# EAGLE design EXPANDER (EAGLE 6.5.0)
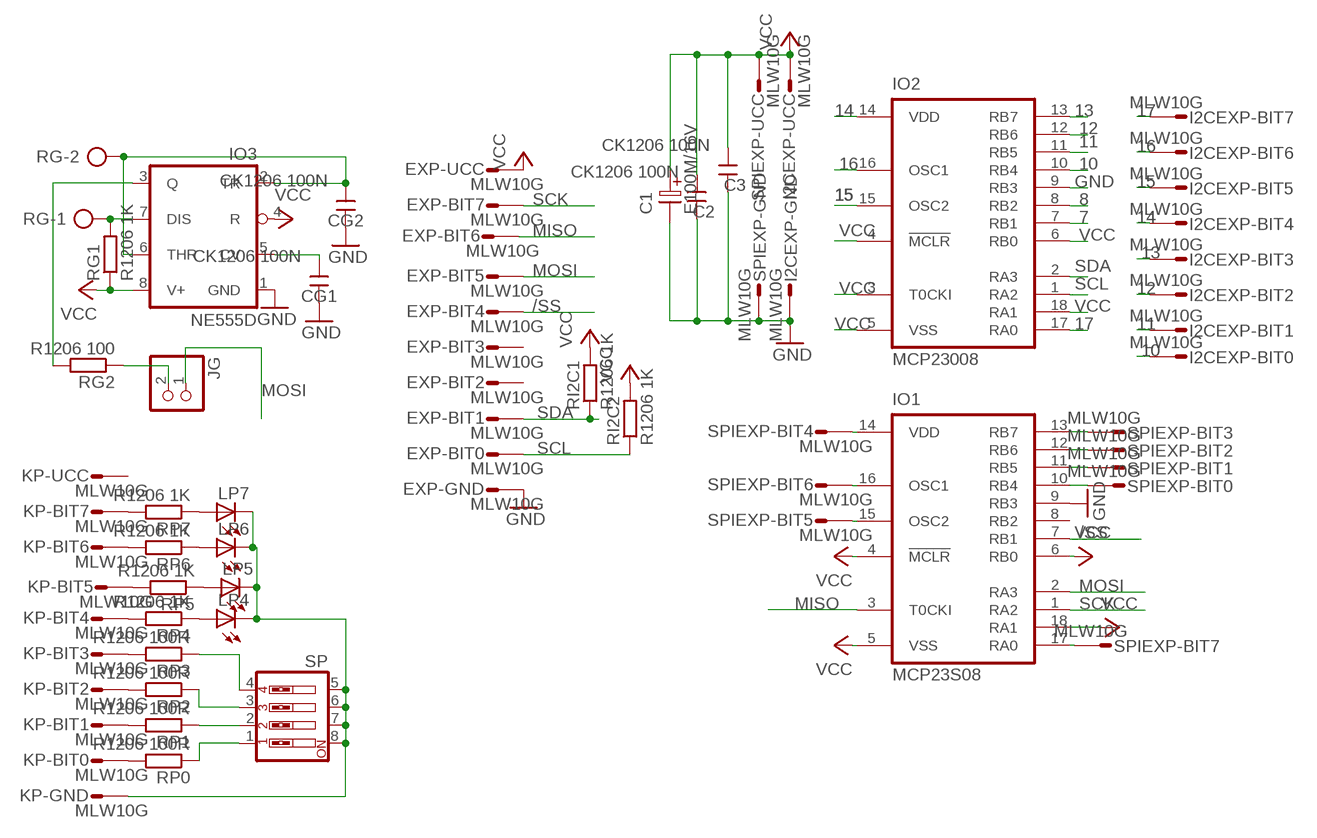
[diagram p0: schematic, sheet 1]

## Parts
C1  E100M/16V  CEL2,5  [ES-2,5L]
C2  CK1206 100N  CK+  [CK+]
C3  CK1206 100N  CK+  [CK+]
CG1  CK1206 100N  CK+  [CK+]
CG2  CK1206 100N  CK+  [CK+]
EXP  MLW10G  PSL10MLW10G  [MLW10G]
I2CEXP  MLW10G  PSL10MLW10G  [MLW10G]
IO1  MCP23S08  PIC16C710SO  [SO-18W]
IO2  MCP23008  PIC16C710SO  [SO-18W]
IO3  NE555D  [SO08]
JG  PINHD-1X2  [1X02]
KP  MLW10G  PSL10MLW10G  [MLW10G]
LP4  LED3MM  [LED3MM]
LP5  LED3MM  [LED3MM]
LP6  LED3MM  [LED3MM]
LP7  LED3MM  [LED3MM]
RG  AK500/2  [AK500/2]
RG1  R1206 1K  R-EU_R1206  [R1206]
RG2  R1206 100  R-EU_R1206  [R1206]
RI2C1  R1206 1K  R-EU_R1206  [R1206]
RI2C2  R1206 1K  R-EU_R1206  [R1206]
RP0  R1206 100R  R-EU_R1206  [R1206]
RP1  R1206 100R  R-EU_R1206  [R1206]
RP2  R1206 100R  R-EU_R1206  [R1206]
RP3  R1206 100R  R-EU_R1206  [R1206]
RP4  R1206 1K  R-EU_R1206  [R1206]
RP5  R1206 1K  R-EU_R1206  [R1206]
RP6  R1206 1K  R-EU_R1206  [R1206]
RP7  R1206 1K  R-EU_R1206  [R1206]
SP  SW_DIP-4  [EDG-04]
SPIEXP  MLW10G  PSL10MLW10G  [MLW10G]
U$1  RAM  [RAM]

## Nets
7: IO2.7(RB1)
8: IO2.8(RB2)
10: I2CEXP.9 IO2.10(RB4)
11: I2CEXP.8 IO2.11(RB5)
12: I2CEXP.7 IO2.12(RB6)
13: I2CEXP.6 IO2.13(RB7)
14: I2CEXP.5 IO2.14(VDD)
15: I2CEXP.4 IO2.15(OSC2)
16: I2CEXP.3 IO2.16(OSC1)
17: I2CEXP.2 IO2.17(RA0)
/SS: EXP.5 IO1.7(RB1)
GND: C1.2 C2.1 C3.1 CG1.1 CG2.1 EXP.10 I2CEXP.10 IO1.9(RB3) IO2.9(RB3) IO3.1(GND) SPIEXP.10
MISO: EXP.3 IO1.3(T0CKI)
MOSI: EXP.4 IO1.2(RA3) JG.1
N$1: KP.10 LP4.K(C) LP5.K(C) LP6.K(C) LP7.K(C) SP.5 SP.6 SP.7 SP.8
N$2: JG.2 RG2.1
N$3: IO1.10(RB4) SPIEXP.9
N$4: IO1.11(RB5) SPIEXP.8
N$6: IO1.12(RB6) SPIEXP.7
N$7: IO1.13(RB7) SPIEXP.6
N$8: IO1.14(VDD) SPIEXP.5
N$9: IO1.15(OSC2) SPIEXP.4
N$10: IO1.16(OSC1) SPIEXP.3
N$11: IO1.17(RA0) SPIEXP.2
N$12: CG1.2 IO3.5(CV)
N$13: IO3.7(DIS) RG1.2 RG.1
N$14: CG2.2 IO3.2(TR) IO3.6(THR) RG.2
N$15: KP.2 RP7.2
N$16: KP.6 RP3.2
N$17: KP.3 RP6.2
N$18: KP.4 RP5.2
N$19: KP.5 RP4.2
N$20: LP7.A RP7.1
N$21: LP6.A RP6.1
N$22: LP5.A RP5.1
N$23: LP4.A RP4.1
N$25: KP.7 RP2.2
N$26: KP.8 RP1.2
N$27: KP.9 RP0.2
N$28: RP3.1 SP.4
N$29: RP2.1 SP.3
N$30: RP1.1 SP.2
N$31: RP0.1 SP.1
PE1: IO3.3(Q) RG2.2
SCK: EXP.2 IO1.1(RA2)
SCL: EXP.9 IO2.1(RA2) RI2C2.1
SDA: EXP.8 IO2.2(RA3) RI2C1.1
VCC: C1.1 C2.2 C3.2 EXP.1 I2CEXP.1 IO1.4(!MCLR) IO1.5(VSS) IO1.6(RB0) IO1.18(RA1) IO2.3(T0CKI) IO2.4(!MCLR) IO2.5(VSS) IO2.6(RB0) IO2.18(RA1) IO3.4(R) IO3.8(V+) RG1.1 RI2C1.2 RI2C2.2 SPIEXP.1
Unconnected: EXP.6 EXP.7 IO1.8(RB2) KP.1

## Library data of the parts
C1 = !MOJE:CEL2,5
C2 C3 CG1 CG2 = !MOJE:CK+
EXP I2CEXP KP SPIEXP = !MOJE:PSL10: CONNECTOR
IO1 IO2 = microchip:PIC16C*: MICROCONTROLLER PIC16C5X family: EPROM/ROM-based PIC16C55X family: EPROM-based PIC16C6X family PIC16CE62X family: analog comparators/EEPROM data memory PIC16C7X family: A/D converter PIC16C71X family: A/D converter PIC16F8X family: flash EEPROM Pin compatible devices: PIC16C154, PIC16CR154,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
IO3 = linear:*555: TIMER
JG = pinhead:PINHD-1X2: PIN HEADER
LP4-LP7 = led:LED: LED
RG = con-ptr500:AK500/2: CONNECTOR; OC_FARNELL: unknown; OC_NEWARK: unknown
RG1 RG2 RI2C1 RI2C2 RP0 RP1-RP7 = rcl:R-EU_: RESISTOR, European symbol
SP = special:SW_DIP-4: DIP SWITCH
U$1 = !MOJE:RAM

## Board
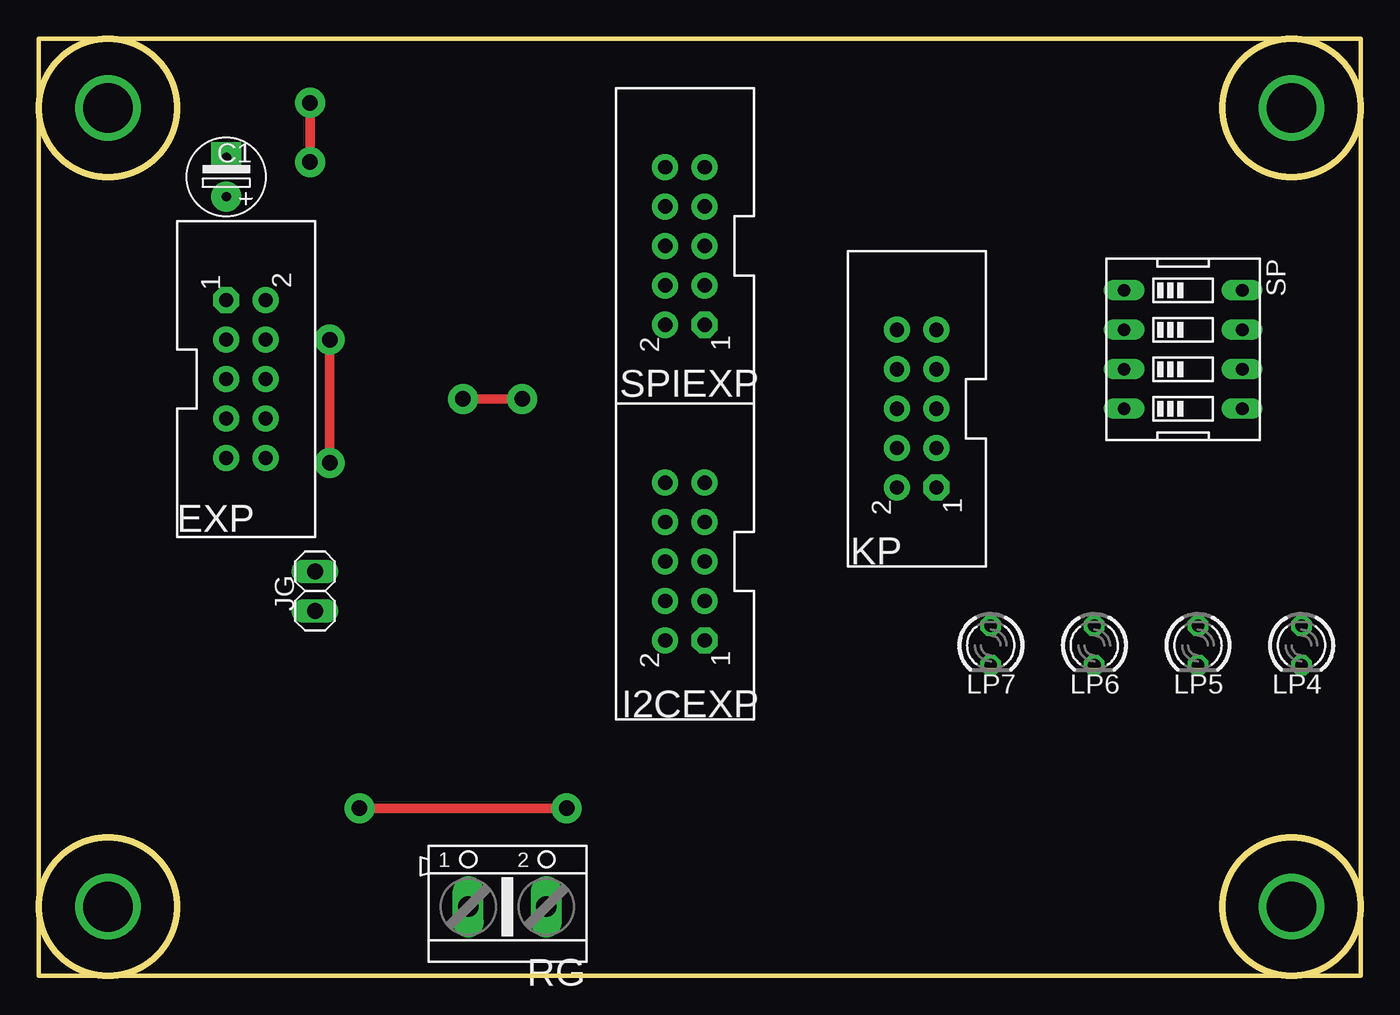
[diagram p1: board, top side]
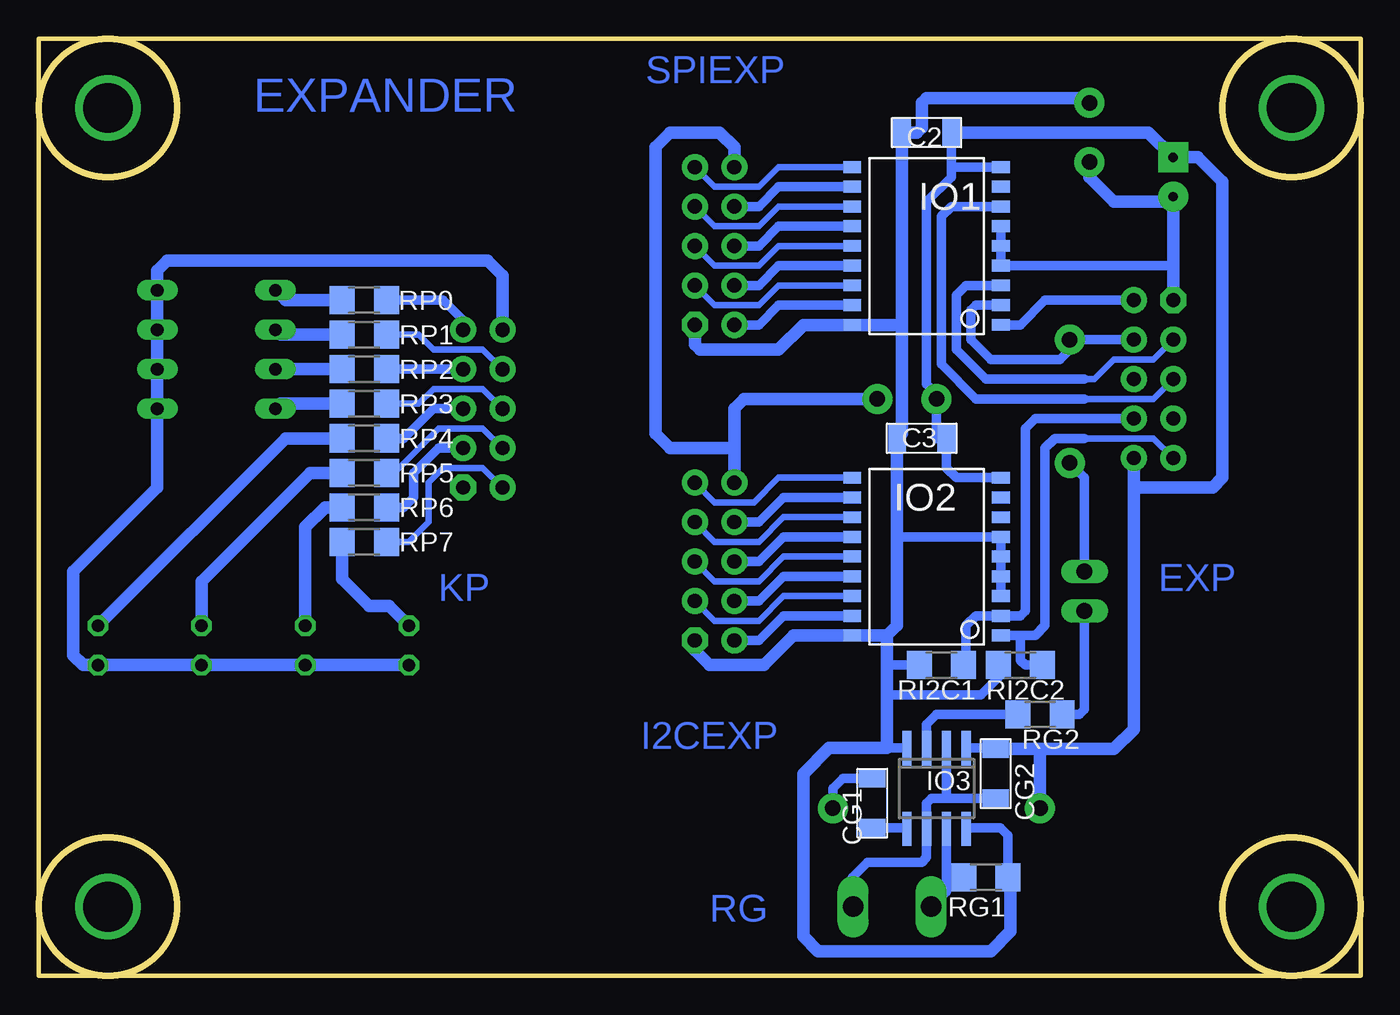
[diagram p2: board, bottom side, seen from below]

Size 85.09 x 60.33 mm. Coordinates in mm from the lower left corner, seen from the top.
Copper layers (1*16): Top 0.035mm / dielectric 1.5mm / Bottom 0.035mm
Design rules "default": minimum track width 10mil, minimum drill 24mil, track to track 8mil, track to pad 8mil, pad to pad 8mil, via to via 8mil, smd to smd 8mil, copper to edge 40mil, drill to drill 8mil, minimum pad ring 10mil, minimum via ring 8mil, stop-mask expansion 4mil, vias tented up to drill 0mil, thermal gap 10mil

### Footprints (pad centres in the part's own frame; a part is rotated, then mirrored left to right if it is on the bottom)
ES-2,5L = drill 0.61 pad 1.93: 1 0,0 | drill 0.61 pad 1.93 square: 2 2.54,0
CK+ = smd 1.14 x 1.7: 1 -1.587,0; 2 1.587,0
MLW10G = drill 0.914 pad 1.676 octagon: 1 -5.08,-1.27 | drill 0.914 pad 1.676: 2 -5.08,1.27; 3 -2.54,-1.27; 4 -2.54,1.27; 5 0,-1.27; 6 0,1.27; 7 2.54,-1.27; 8 2.54,1.27; 9 5.08,-1.27; 10 5.08,1.27
SO-18W = smd 0.762 x 1.143: 1 -5.08,-4.788; 2 -3.81,-4.788; 3 -2.54,-4.788; 4 -1.27,-4.788; 5 0,-4.788; 6 1.27,-4.788; 7 2.54,-4.788; 8 3.81,-4.788; 9 5.08,-4.788; 10 5.08,4.788; 11 3.81,4.788; 12 2.54,4.788; 13 1.27,4.788; 14 0,4.788; 15 -1.27,4.788; 16 -2.54,4.788; 17 -3.81,4.788; 18 -5.08,4.788
SO08 = smd 0.6 x 2.2: 1 -1.905,-2.6; 2 -0.635,-2.6; 3 0.635,-2.6; 4 1.905,-2.6; 5 1.905,2.6; 6 0.635,2.6; 7 -0.635,2.6; 8 -1.905,2.6
1X02 = drill 1.016 long: 1 -1.27,0; 2 1.27,0
LED3MM = drill 0.813 octagon: A -1.27,0; K 1.27,0
AK500/2 = drill 1.321 long: 1 -2.515,0; 2 2.515,0
R1206 = smd 1.6 x 1.803: 1 -1.422,0; 2 1.422,0
EDG-04 = drill 0.813 long: 1 -3.81,-3.81; 2 -1.27,-3.81; 3 1.27,-3.81; 4 3.81,-3.81; 5 3.81,3.81; 6 1.27,3.81; 7 -1.27,3.81; 8 -3.81,3.81
RAM = drill 3.2: P$1 -37.465,-26.035; P$2 -37.465,25.4; P$3 38.735,25.4; P$4 38.735,-26.035

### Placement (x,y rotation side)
C1  12.07,50.16 90 top
C2  27.94,54.29 180 bottom
C3  28.26,34.61 180 bottom
CG1  31.43,11.11 270 bottom
CG2  23.5,13.02 270 bottom
EXP  13.34,38.42 270 top
I2CEXP  41.59,26.67 90 top
IO1  27.94,46.99 90 bottom
IO2  27.94,26.99 90 bottom
IO3  27.31,12.06 180 bottom
JG  17.78,24.77 270 top
KP  56.52,36.51 90 top
LP4  81.28,21.27 270 top
LP5  74.61,21.27 270 top
LP6  67.94,21.27 270 top
LP7  61.28,21.27 270 top
RG  30.16,4.45 0 top
RG1  24.13,6.35 180 bottom
RG2  20.64,16.83 180 bottom
RI2C1  26.99,20 180 bottom
RI2C2  21.91,20 180 bottom
RP0  64.14,43.5 0 bottom
RP1  64.14,41.27 0 bottom
RP2  64.14,39.05 0 bottom
RP3  64.14,36.83 0 bottom
RP4  64.14,34.61 0 bottom
RP5  64.14,32.38 0 bottom
RP6  64.14,30.16 0 bottom
RP7  64.14,27.94 0 bottom
SP  73.66,40.32 270 top
SPIEXP  41.59,46.99 90 top
U$1  41.91,30.48 0 top

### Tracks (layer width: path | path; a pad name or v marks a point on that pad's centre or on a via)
10
  Bottom 0.406: IO2.10 37.47,32.07 39.05,30.48 41.59,30.48 I2CEXP.9
11
  Bottom 0.61: IO2.11 37.15,30.8 38.74,29.21 I2CEXP.8
12
  Bottom 0.406: IO2.12 37.15,29.53 38.74,27.94 41.59,27.94 I2CEXP.7
13
  Bottom 0.61: IO2.13 37.15,28.26 38.74,26.67 I2CEXP.6
14
  Bottom 0.406: IO2.14 37.15,26.99 38.74,25.4 41.59,25.4 I2CEXP.5
15
  Bottom 0.61: IO2.15 37.15,25.72 38.74,24.13 I2CEXP.4
16
  Bottom 0.406: IO2.16 37.15,24.45 38.74,22.86 41.59,22.86 I2CEXP.3
17
  Bottom 0.61: IO2.17 37.15,23.18 38.74,21.59 I2CEXP.2
/SS
  Bottom 0.406: EXP.5 13.34,37.15 17.78,37.15
  Bottom 0.61: 17.78,37.15 24.77,37.15 26.99,39.37 26.99,48.9 26.35,49.53 IO1.7
GND  (via drill 1 pad 1.93)
  Top 0.61: v31.12,37.15 v27.31,37.15 | v33.97,10.79 v20.64,10.79
  Bottom 0.406: 23.56,14.66 CG2.1
  Bottom 0.61: C2.1 26.35,52.07 | 26.35,52.07 26.35,51.44 27.94,49.85 27.94,38.1 27.31,37.47 v27.31,37.15 27.31,34.61 C3.1 26.67,32.7 26.04,32.07 IO2.9 | IO1.9 26.35,52.07 | IO3.1 23.56,14.66 | CG1.1 33.34,12.7 33.97,12.06 v33.97,10.79 | 20.64,14.29 20.32,14.61
  Bottom 0.813: EXP.10 14.61,31.43 | 14.61,31.43 9.53,31.43 8.89,32.07 8.89,51.12 10.48,52.7 C1.2 13.65,54.29 C2.1 | I2CEXP.10 40.32,33.97 | 40.32,33.97 40.32,36.51 39.69,37.15 v31.12,37.15 | SPIEXP.10 40.32,53.34 41.28,54.29 44.45,54.29 45.4,53.34 45.4,34.92 44.45,33.97 40.32,33.97 | CG2.1 20.32,14.61 15.88,14.61 14.61,15.88 14.61,31.43 | v20.64,10.79 20.64,14.29
MISO
  Bottom 0.406: EXP.3 13.34,39.69 15.88,39.69 17.15,38.42 17.78,38.42
  Bottom 0.61: 17.78,38.42 24.13,38.42 26.04,40.32 26.04,43.81 25.4,44.45 IO1.3
MOSI  (via drill 1 pad 1.93)
  Top 0.61: v18.73,33.02 v18.73,40.96
  Bottom 0.61: JG.1 17.78,32.07 v18.73,33.02 | EXP.4 v18.73,40.96 18.73,40.32 19.37,39.69 23.81,39.69 25.08,40.96 25.08,42.86 24.77,43.18 IO1.2
N$1
  Bottom 0.813: LP7.K LP6.K LP5.K | LP5.K LP4.K | LP5.K 82.23,20 82.87,20.64 82.87,26.04 77.47,31.43 SP.5 SP.6 SP.7 SP.8 77.47,45.4 76.84,46.04 56.2,46.04 55.25,45.09 KP.10
N$2
  Bottom 0.61: JG.2 17.78,17.14 18.1,16.83 RG2.1
N$3
  Bottom 0.406: IO1.10 37.47,52.07 38.74,50.8 41.59,50.8 SPIEXP.9
N$4
  Bottom 0.61: IO1.11 37.47,50.8 38.74,49.53 SPIEXP.8
N$6
  Bottom 0.406: IO1.12 37.47,49.53 38.74,48.26 41.59,48.26 SPIEXP.7
N$7
  Bottom 0.61: IO1.13 37.47,48.26 38.74,46.99 SPIEXP.6
N$8
  Bottom 0.406: IO1.14 37.47,46.99 38.74,45.72 41.59,45.72 SPIEXP.5
N$9
  Bottom 0.61: IO1.15 37.47,45.72 38.74,44.45 SPIEXP.4
N$10
  Bottom 0.406: IO1.16 37.47,44.45 38.74,43.18 41.59,43.18 SPIEXP.3
N$11
  Bottom 0.61: IO1.17 37.47,43.18 38.74,41.91 SPIEXP.2
N$12
  Bottom 0.61: CG1.2 29.27,9.53 IO3.5
N$13
  Bottom 0.61: IO3.7 26.67,6.35 | 26.67,6.35 26.67,5.42 RG.1 | RG1.2 26.67,6.35
N$14
  Bottom 0.406: 26.67,11.75 26.35,11.43 | 32.7,4.47 RG.2
  Bottom 0.61: CG2.2 26.35,11.43 27.62,11.43 27.94,11.11 IO3.6 27.94,7.62 28.26,7.3 31.75,7.3 32.7,6.35 32.7,4.47 | IO3.2 26.67,11.75
N$15
  Bottom 0.406: KP.2 56.52,32.7 59.06,32.7 60.01,31.75 60.01,29.21 61.28,27.94 RP7.2
N$16
  Bottom 0.406: KP.6 56.52,37.78 59.69,37.78 60.64,36.83 RP3.2
N$17
  Bottom 0.61: KP.3 59.37,33.97 60.96,32.38 60.96,30.8 61.6,30.16 RP6.2
N$18
  Bottom 0.406: KP.4 56.52,35.24 59.37,35.24 62.23,32.38 RP5.2
N$19
  Bottom 0.61: KP.5 59.69,36.51 61.6,34.61 RP4.2
N$20
  Bottom 0.813: RP7.1 65.56,25.55 63.82,23.81 62.55,23.81 LP7.A
N$21
  Bottom 0.813: RP6.1 66.68,30.16 67.94,28.89 LP6.A
N$22
  Bottom 0.813: RP5.1 67.63,32.38 74.61,25.4 LP5.A
N$23
  Bottom 0.813: RP4.1 69.22,34.61 LP4.A
N$25
  Bottom 0.61: KP.7 RP2.2
N$26
  Bottom 0.406: KP.8 56.52,40.32 59.69,40.32 60.64,41.27 RP1.2
N$27
  Bottom 0.61: KP.9 57.79,42.23 59.06,43.5 RP0.2
N$28
  Bottom 0.813: RP3.1 69.53,36.83 SP.4
N$29
  Bottom 0.813: SP.3 RP2.1
N$30
  Bottom 0.813: RP1.1 69.53,41.27 SP.2
N$31
  Bottom 0.813: RP0.1 69.22,43.5 SP.1
PE1
  Bottom 0.61: RG2.2 27.31,16.83 27.94,16.19 IO3.3
SCK
  Bottom 0.61: EXP.2 20.32,43.5 21.91,41.91 IO1.1
SCL
  Bottom 0.406: EXP.9 13.34,34.61 17.78,34.61
  Bottom 0.61: 17.78,34.61 19.69,34.61 20.32,33.97 20.32,22.54 20.96,21.91 21.91,21.91 | 21.91,21.91 IO2.1 | RI2C2.1 21.59,20 21.91,20.32 21.91,21.91
SDA
  Bottom 0.61: EXP.8 20.96,35.88 21.59,35.24 21.59,23.5 21.91,23.18 IO2.2 24.77,23.18 25.4,22.54 25.4,20.17 RI2C1.1
VCC  (via drill 1 pad 1.93)
  Top 0.61: v17.46,56.2 v17.46,52.39
  Bottom 0.406: 29.53,34.92 C3.2 | 12.07,45.72 EXP.1 | 25.34,9.53 IO3.8 | 22.54,6.18 RG1.1
  Bottom 0.61: IO1.6 IO1.5 IO1.4 12.07,45.72 | 29.85,28.26 IO2.6 IO2.5 IO2.4 IO2.3 | 12.38,49.85 C1.1 | RG1.1 22.71,9.06 23.18,9.53 25.34,9.53 | IO3.4 30.48,14.66 | RI2C1.2 30.48,20 | RI2C2.2 23.33,19.21 24.45,18.1 30.48,18.1
  Bottom 0.813: 29.53,41.91 C2.2 28.58,54.29 28.26,54.61 28.26,56.2 27.94,56.52 17.78,56.52 v17.46,56.2 | 29.53,41.91 IO1.18 35.88,41.91 37.47,40.32 42.55,40.32 42.86,40.64 SPIEXP.1 | 29.53,41.91 29.53,34.92 | C3.2 29.85,28.26 29.85,22.54 30.48,21.91 | 30.48,21.91 IO2.18 36.51,21.91 38.42,20 41.91,20 42.86,20.95 I2CEXP.1 | EXP.1 C1.1 | v17.46,52.39 17.46,51.44 15.88,49.85 12.38,49.85 | 22.54,6.18 22.54,2.86 23.81,1.59 34.93,1.59 35.88,2.54 35.88,13.02 34.23,14.66 30.48,14.66 30.48,18.1 30.48,20 30.48,21.91

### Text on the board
Bottom: EXPANDER | SPIEXP | EXP | KP | I2CEXP | RG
